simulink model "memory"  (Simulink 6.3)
settings: Solver=ode45  StartTime=0.0  StopTime=25.0  RelTol=1e-3
undefined symbols (not defined in the file or in its folder): Bit, Location, Lower, netlist, Width
libraries: xbsIndex_r4 x22, adlibrary2 x2

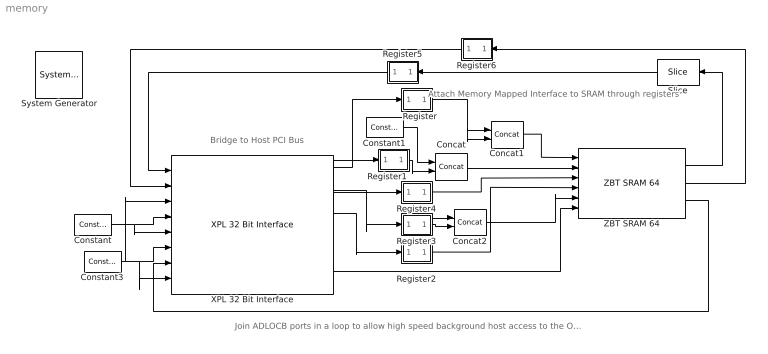
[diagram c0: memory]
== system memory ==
  note: Bridge to Host PCI Bus
  note: Attach Memory Mapped Interface to SRAM through registers
  note: Join ADLOCB ports in a loop to allow high speed background host access to the Off Chip Ram
  " System Generator" : xbsIndex_r4/ System Generator  Tag=genX  xilinxfamily=Virtex2P  part=xc2vp30  speed=-6  package=ff896  synthesis_tool=XST  directory=./netlist  testbench=off  simulink_period=1  sysclk_period=7.5  incr_netlist=off  trim_vbits=Everywhere in SubSystem  dbl_ovrd=According to Block Masks  core_generation=According to Block Masks  run_coregen=off  deprecated_control=off  eval_field=0  block_type=sysgen
  Concat : xbsIndex_r4/Concat  num_inputs=2  dbl_ovrd=off  block_type=concat
  Concat1 : xbsIndex_r4/Concat  num_inputs=2  dbl_ovrd=off  block_type=concat
  Concat2 : xbsIndex_r4/Concat  num_inputs=2  dbl_ovrd=off  block_type=concat
  Constant : xbsIndex_r4/Constant  arith_type=Boolean  const=0  n_bits=1  bin_pt=0  explicit_period=on  period=1  equ=P=C  opselect=C  inp2=PCIN>>17  opr=+  inp1=P  carry=CIN  dbl_ovrd=off  block_type=constant
  Constant1 : xbsIndex_r4/Constant  arith_type=Unsigned  const=0  n_bits=4  bin_pt=0  explicit_period=on  period=1  equ=P=C  opselect=C  inp2=PCIN>>17  opr=+  inp1=P  carry=CIN  dbl_ovrd=off  block_type=constant
  Constant3 : xbsIndex_r4/Constant  arith_type=Unsigned  const=0  n_bits=32  bin_pt=0  explicit_period=on  period=1  equ=P=C  opselect=C  inp2=PCIN>>17  opr=+  inp1=P  carry=CIN  dbl_ovrd=off  block_type=constant
  Register : Subsystem
  Register1 : Subsystem
  Register2 : Subsystem
  Register3 : Subsystem
  Register4 : Subsystem
  Register5 : Subsystem  Orientation=left
  Register6 : Subsystem  Orientation=left
  Slice : xbsIndex_r4/Slice  Orientation=left  nbits=32  boolean_output=off  mode=Lower Bit Location + Width  bit1=0  base1=MSB of Input  bit0=0  base0=LSB of Input  dbl_ovrd=off  block_type=slice
  XPL 32 Bit Interface : adlibrary2/ADM-XPL/XPL 32 Bit Interface  program='slave_write 0x0 0x1234;slave_read 0x0'  clock_ratio=1.5
  ZBT SRAM 64 : adlibrary2/ADM-XPL/ZBT SRAM 64
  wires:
  Constant/1 -> XPL 32 Bit Interface/5, XPL 32 Bit Interface/4
  Constant3/1 -> XPL 32 Bit Interface/3, XPL 32 Bit Interface/6, XPL 32 Bit Interface/8
  XPL 32 Bit Interface/5 -> Register2/1(in0)
  XPL 32 Bit Interface/2 -> Register1/1(in0)
  XPL 32 Bit Interface/1 -> Register/1(in0)
  XPL 32 Bit Interface/10 -> ZBT SRAM 64/6
  ZBT SRAM 64/3 -> XPL 32 Bit Interface/7
  ZBT SRAM 64/2 -> Register6/1(in0)
  ZBT SRAM 64/1 -> Slice/1
  Register/1(out0) -> Concat1/2, Concat1/1
  Register2/1(out0) -> ZBT SRAM 64/4
  Register4/1(out0) -> ZBT SRAM 64/3
  Concat/1 -> ZBT SRAM 64/2
  Constant1/1 -> Concat/1
  Register1/1(out0) -> Concat/2
  Register5/1(out0) -> XPL 32 Bit Interface/1
  Register6/1(out0) -> XPL 32 Bit Interface/2
  Concat1/1 -> ZBT SRAM 64/1
  Register3/1(out0) -> Concat2/1, Concat2/2
  Concat2/1 -> ZBT SRAM 64/5
  Slice/1 -> Register5/1(in0)
  XPL 32 Bit Interface/4 -> Register4/1(in0)
  XPL 32 Bit Interface/3 -> Register3/1(in0)

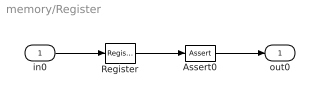
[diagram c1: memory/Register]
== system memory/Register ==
  in0 : Inport
  Assert0 : xbsIndex_r4/Assert  assert_type=off  type_source=Explicitly  arith_type="Signed  (2's comp)"  n_bits=16  bin_pt=14  assert_rate=on  rate_source=Explicitly  period=1  output_port=on  block_type=assert
  Register : xbsIndex_r4/Register  init=0  rst=off  en=off  dbl_ovrd=off  block_type=register
  out0 : Outport
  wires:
  in0/1 -> Register/1
  Register/1 -> Assert0/1
  Assert0/1 -> out0/1

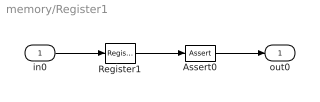
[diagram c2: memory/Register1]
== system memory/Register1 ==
  in0 : Inport
  Assert0 : xbsIndex_r4/Assert  assert_type=off  type_source=Explicitly  arith_type="Signed  (2's comp)"  n_bits=16  bin_pt=14  assert_rate=on  rate_source=Explicitly  period=1  output_port=on  block_type=assert
  Register1 : xbsIndex_r4/Register  init=0  rst=off  en=off  dbl_ovrd=off  block_type=register
  out0 : Outport
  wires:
  in0/1 -> Register1/1
  Register1/1 -> Assert0/1
  Assert0/1 -> out0/1

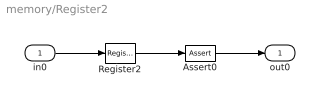
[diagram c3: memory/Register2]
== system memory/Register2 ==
  in0 : Inport
  Assert0 : xbsIndex_r4/Assert  assert_type=off  type_source=Explicitly  arith_type="Signed  (2's comp)"  n_bits=16  bin_pt=14  assert_rate=on  rate_source=Explicitly  period=1  output_port=on  block_type=assert
  Register2 : xbsIndex_r4/Register  init=0  rst=off  en=off  dbl_ovrd=off  block_type=register
  out0 : Outport
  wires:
  in0/1 -> Register2/1
  Register2/1 -> Assert0/1
  Assert0/1 -> out0/1

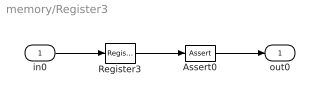
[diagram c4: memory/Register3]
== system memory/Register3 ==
  in0 : Inport
  Assert0 : xbsIndex_r4/Assert  assert_type=off  type_source=Explicitly  arith_type="Signed  (2's comp)"  n_bits=16  bin_pt=14  assert_rate=on  rate_source=Explicitly  period=1  output_port=on  block_type=assert
  Register3 : xbsIndex_r4/Register  init=0  rst=off  en=off  dbl_ovrd=off  block_type=register
  out0 : Outport
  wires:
  in0/1 -> Register3/1
  Register3/1 -> Assert0/1
  Assert0/1 -> out0/1

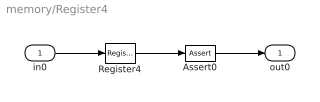
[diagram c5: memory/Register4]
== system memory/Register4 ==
  in0 : Inport
  Assert0 : xbsIndex_r4/Assert  assert_type=off  type_source=Explicitly  arith_type="Signed  (2's comp)"  n_bits=16  bin_pt=14  assert_rate=on  rate_source=Explicitly  period=1  output_port=on  block_type=assert
  Register4 : xbsIndex_r4/Register  init=0  rst=off  en=off  dbl_ovrd=off  block_type=register
  out0 : Outport
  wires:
  in0/1 -> Register4/1
  Register4/1 -> Assert0/1
  Assert0/1 -> out0/1

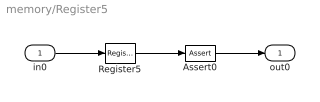
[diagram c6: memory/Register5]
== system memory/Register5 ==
  in0 : Inport
  Assert0 : xbsIndex_r4/Assert  assert_type=off  type_source=Explicitly  arith_type="Signed  (2's comp)"  n_bits=16  bin_pt=14  assert_rate=on  rate_source=Explicitly  period=1  output_port=on  block_type=assert
  Register5 : xbsIndex_r4/Register  init=0  rst=off  en=off  dbl_ovrd=off  block_type=register
  out0 : Outport
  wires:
  in0/1 -> Register5/1
  Register5/1 -> Assert0/1
  Assert0/1 -> out0/1

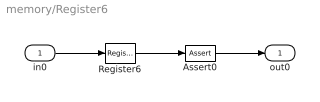
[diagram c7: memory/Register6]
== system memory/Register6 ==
  in0 : Inport
  Assert0 : xbsIndex_r4/Assert  assert_type=off  type_source=Explicitly  arith_type="Signed  (2's comp)"  n_bits=16  bin_pt=14  assert_rate=on  rate_source=Explicitly  period=1  output_port=on  block_type=assert
  Register6 : xbsIndex_r4/Register  init=0  rst=off  en=off  dbl_ovrd=off  block_type=register
  out0 : Outport
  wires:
  in0/1 -> Register6/1
  Register6/1 -> Assert0/1
  Assert0/1 -> out0/1
